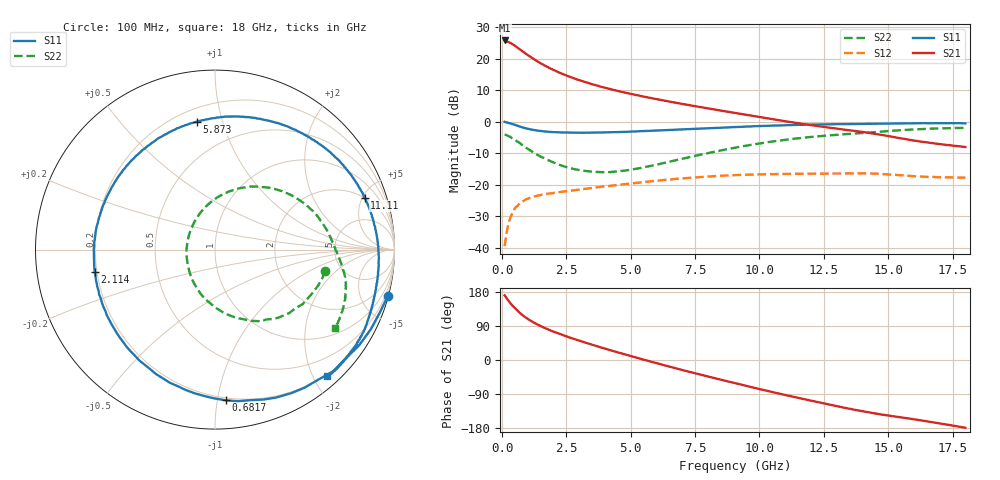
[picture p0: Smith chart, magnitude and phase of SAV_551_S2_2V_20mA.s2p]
! Data provided by Modelithics, Inc.  Tampa, Florida USA, June 2008
!Model SAV-551+
!VAR V_out= 2
!VAR I_out= 20
!VAR V_in= 0.3569
!VAR I_in= 0.9437
!BEGIN ACDATA
# GHZ S MA R 50
! Scattering Parameters
!% F n11x n11y n21x n21y n12x n12y n22x n22y
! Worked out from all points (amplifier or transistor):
!   401 points, 100 MHz to 18 GHz, reference 50 ohm
!   highest |S21| = 25.9 dB at 100 MHz (marker M1)
!   |S21| within 3 dB of that: start of sweep to 718.4 MHz
!   unconditionally stable (mu >= 1): 4.36 GHz to 10.7 GHz; 10.71 GHz to 10.89 GHz
!   at 3.054 GHz: K = 0.84, MSG = 17.3 dB, |S12| = -21.6 dB
!   at 9.05 GHz: K = 1.06, MAG = 8.4 dB, |S12| = -17.0 dB
!   at 18 GHz: K = 0.90, MSG = 4.9 dB, |S12| = -17.7 dB
!   lowest NFmin = 0.09 dB at 500 MHz
!   S11 on the Smith chart (normalised r, x): 100 MHz: 0.09, -7.62; 681.8 MHz: 0.18, -1.06; 2.114 GHz: 0.19, -0.09; 5.873 GHz: 0.28, +0.83; 11.11 GHz: 2.00, +5.19; 18 GHz: 0.17, -2.20
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0.1  0.9968 -14.9  19.62 170.7  0.01051 80.1  0.6218 -11.0
0.1895  0.9748 -27.1  18.85 162.0  0.0182 76.0  0.61 -18.7
0.32375  0.9452 -45.9  17.95 150.1  0.03029 67.1  0.5752 -31.9
0.41325  0.917 -57.0  17.05 142.7  0.03574 60.2  0.5445 -40.4
0.5475  0.8778 -72.1  15.64 133.3  0.04434 53.4  0.5017 -50.5
0.68175  0.842 -85.8  14.26 124.8  0.04979 46.5  0.4596 -60.1
0.816  0.8087 -98.0  12.98 117.2  0.05442 42.0  0.4172 -68.2
0.95025  0.783 -108.9  11.87 110.6  0.05905 37.9  0.3829 -75.9
1.0845  0.7578 -118.4  10.85 104.7  0.06158 34.3  0.3519 -82.8
1.2635  0.7358 -129.9  9.733 97.7  0.06506 30.3  0.3162 -91.1
1.6215  0.7047 -148.8  7.976 85.7  0.06992 24.5  0.2652 -106.1
2.11375  0.6816 -169.3  6.344 71.9  0.0747 19.0  0.2151 -124.4
3.09825  0.6691 159.6  4.44 48.9  0.08428 10.6  0.1678 -157.8
4.396  0.6836 127.9  3.16 22.1  0.09771 0.8  0.161 159.7
5.87275  0.7192 98.1  2.343 -6.0  0.1139 -12.0  0.2016 120.5
6.0965  0.7271 94.1  2.251 -10.0  0.1161 -13.9  0.2122 115.6
7.439  0.7693 71.3  1.785 -33.9  0.1294 -27.3  0.2834 89.6
9.05  0.8219 47.2  1.377 -61.0  0.1416 -44.2  0.3867 63.8
11.1085  0.8817 19.1  1.004 -94.0  0.148 -67.2  0.5248 35.1
12.04825  0.9005 7.6  0.8781 -107.9  0.1494 -77.6  0.576 23.7
15.0465  0.936 -23.6  0.5876 -147.0  0.1452 -107.7  0.7125 -7.2
18  0.9423 -48.6  0.3967 -178.7  0.1296 -132.8  0.7981 -33.0
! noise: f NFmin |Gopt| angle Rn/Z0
0.5  0.092  0.2135  54.21  0.069
0.7  0.129  0.2385  61.64  0.062
0.9  0.166  0.2623  69.07  0.055
1  0.185  0.2738  72.78  0.053
1.9  0.351  0.3647  106.1  0.036
2.4  0.444  0.4053  124.7  0.033
3  0.555  0.4446  146.8  0.037
3.9  0.722  0.4846  180  0.056
5  0.926  0.5023  -139.6  0.1
6  1.111  0.4888  -102.9  0.161
